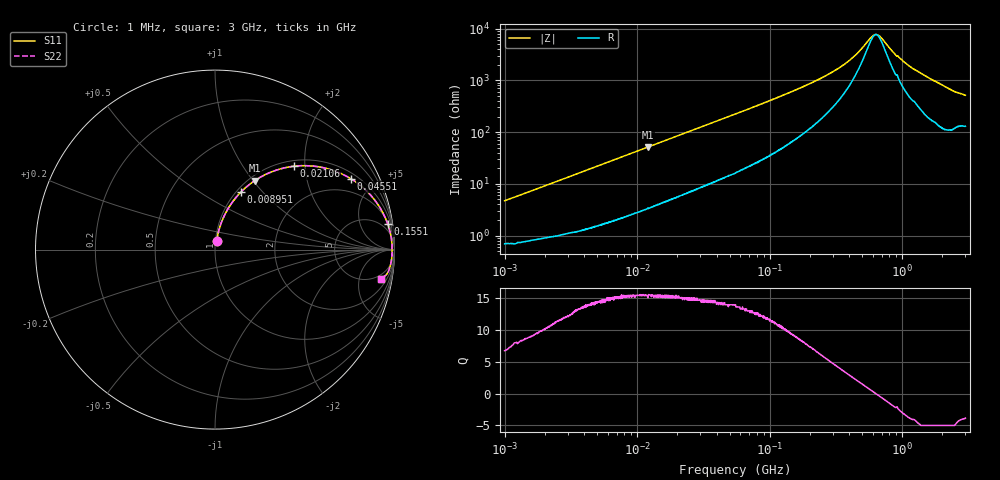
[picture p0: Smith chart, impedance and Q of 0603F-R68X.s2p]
!s-Parameter Generated by FASTRON Sdn. Bhd.
!FASTRON P/N : 0603F-R68X
!Keysight Technologies: E4991B_MY54100416_A.01.15
!Date: Thu Jun 20 13:33:18 2024
!Version  :Rev00  Thu Jun 20 13:33:18 2024
!Data & Calibration Information:
!Freq  S11  S21  S12  S22
!PortZ  Port1:50+j0  Port2:50+j0
!When reading reference impedance value at option line is always used.
! Remarks : This data is being provided solely for informational purposes.
# Hz S dB R 50
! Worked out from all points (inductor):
!   1601 points, 1 MHz to 3 GHz, reference 50 ohm
!   read as one part in series: L = 732 nH near 1.041 MHz
!   highest Q = 15.5 at 12.02 MHz (marker M1), where L = 677 nH
!   self-resonance near 633.9 MHz
!   S11 on the Smith chart (normalised r, x): 1 MHz: 1.01, +0.09; 8.951 MHz: 1.05, +0.77; 21.06 MHz: 1.12, +1.76; 45.51 MHz: 1.26, +3.70; 155.1 MHz: 2, +13; 3 GHz: 4, -10
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1000000  -26.60 78.9  -0.07 -2.6  -0.07 -2.6  -26.60 78.9
3804036  -15.70 76.3  -0.23 -9.4  -0.23 -9.4  -15.70 76.3
8950802  -9.07 65.7  -0.79 -20.6  -0.79 -20.6  -9.07 65.7
1.202488e7  -7.04 59.9  -1.24 -26.3  -1.24 -26.3  -7.04 59.9
1.447069e7  -5.88 55.8  -1.63 -30.5  -1.63 -30.5  -5.88 55.8
2.106101e7  -3.88 46.5  -2.77 -39.7  -2.77 -39.7  -3.88 46.5
3.03475e7  -2.42 37.1  -4.38 -49.0  -4.38 -49.0  -2.42 37.1
4.551475e7  -1.36 27.4  -6.73 -58.6  -6.73 -58.6  -1.36 27.4
5.504702e7  -1.02 23.4  -8.01 -62.5  -8.01 -62.5  -1.02 23.4
8.723049e7  -0.52 15.4  -11.50 -69.9  -11.50 -69.9  -0.52 15.4
1.550909e8  -0.24 8.6  -16.50 -75.1  -16.50 -75.1  -0.24 8.6
2.083556e8  -0.18 6.1  -19.30 -75.9  -19.30 -75.9  -0.18 6.1
2.884452e8  -0.14 4.0  -23.00 -74.7  -23.00 -74.7  -0.14 4.0
3.779341e8  -0.12 2.5  -26.90 -70.4  -26.90 -70.4  -0.12 2.5
4.548043e8  -0.12 1.6  -30.40 -62.8  -30.40 -62.8  -0.12 1.6
6.140682e8  -0.11 0.1  -37.70 -11.2  -37.70 -11.2  -0.11 0.1
6.753166e8  -0.11 -0.3  -37.30 21.5  -37.30 21.5  -0.11 -0.3
7.925923e8  -0.11 -1.1  -33.00 54.0  -33.00 54.0  -0.11 -1.1
8.804142e8  -0.12 -1.6  -30.30 63.2  -30.30 63.2  -0.12 -1.6
1.206698e9  -0.14 -3.2  -24.70 72.9  -24.70 72.9  -0.14 -3.2
2.324278e9  -0.30 -8.2  -16.80 72.2  -16.80 72.2  -0.30 -8.2
3e9  -0.55 -10.1  -14.80 65.3  -14.80 65.3  -0.55 -10.1
